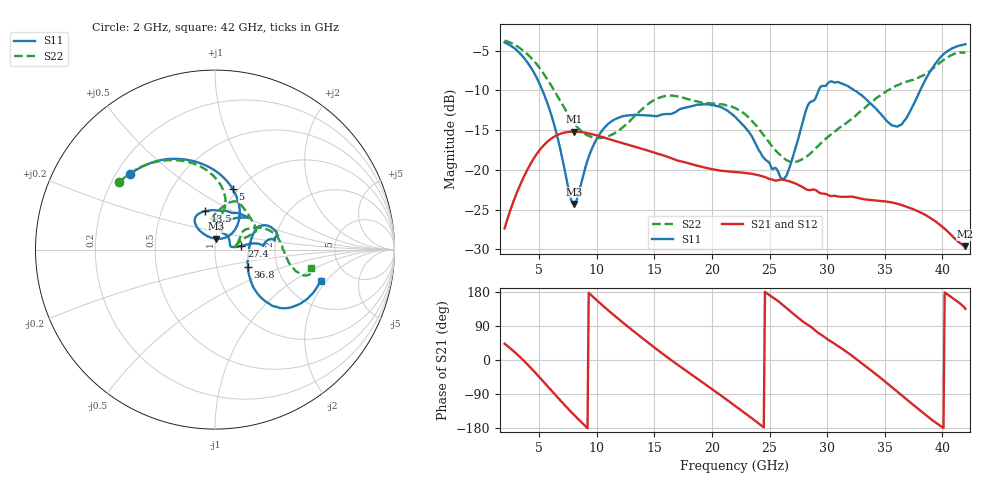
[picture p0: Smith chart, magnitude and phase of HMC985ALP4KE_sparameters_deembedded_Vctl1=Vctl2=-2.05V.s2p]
!s2p File: Measurements: S11, S21, S12, S22
# GHz S dB R 50.0
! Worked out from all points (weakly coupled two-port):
!   401 points, 2 GHz to 42 GHz, reference 50 ohm
!   highest |S21| = -15.18 dB at 8 GHz (marker M1); lowest = -29.6 dB at 42 GHz (marker M2)
!   lowest |S11| = -24.3 dB at 8 GHz (marker M3), VSWR 1.13, Z = 50.3 + j6.11 ohm
!   |S11| at or under -10 dB: 5.285 GHz to 29.26 GHz (23.98 GHz wide, 139 % of centre); 32.37 GHz to 38.07 GHz (5.705 GHz wide, 16.2 % of centre)
!   |S22| runs from -19.0 to -3.7 dB; largest |S21 - S12| = 0.00019
!   S11 on the Smith chart (normalised r, x): 2 GHz: 0.25, +0.36; 5 GHz: 0.94, +0.73; 13.5 GHz: 0.82, +0.37; 27.4 GHz: 1.34, +0.06; 36.8 GHz: 1.41, -0.29; 42 GHz: 3.16, -1.78
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2  -3.96 138.4  -27.37 42.9  -27.38 42.9  -3.72 144.9
3.5  -5.61 107.4  -21.40 3.0  -21.41 3.0  -4.87 119.6
5  -9.05 73.8  -17.59 -44.6  -17.59 -44.6  -7.10 95.5
6.6  -15.95 45.1  -15.61 -98.8  -15.61 -98.8  -10.75 78.5
8  -24.30 83.8  -15.18 -144.1  -15.19 -144.1  -14.04 79.9
8.7  -21.39 119.2  -15.26 -165.3  -15.26 -165.3  -15.18 86.2
10.6  -14.81 127.2  -15.92 141.4  -15.93 141.4  -15.93 100.1
13.5  -13.08 104.7  -17.17 68.7  -17.18 68.7  -12.95 83.3
15.4  -13.18 80.5  -18.02 23.9  -18.02 23.9  -10.93 70.2
18.9  -11.81 44.5  -19.54 -52.8  -19.55 -52.7  -11.45 44.9
22  -13.31 54.9  -20.27 -120.7  -20.28 -120.7  -12.22 23.5
24.5  -18.48 77.3  -20.86 -177.8  -20.86 -177.8  -15.64 20.1
26.1  -21.17 17.9  -21.24 146.5  -21.24 146.5  -18.38 11.7
27.4  -16.58 8.0  -21.82 113.4  -21.82 113.3  -18.97 8.3
28.7  -11.36 4.4  -22.49 84.9  -22.50 84.9  -17.70 15.7
29.5  -9.48 9.1  -22.97 66.2  -22.98 66.2  -16.58 23.2
31.1  -9.05 16.9  -23.38 33.7  -23.38 33.6  -14.67 33.0
33.3  -11.01 27.7  -23.72 -15.2  -23.73 -15.2  -12.16 29.3
35.4  -14.13 7.9  -24.06 -66.1  -24.05 -66.1  -9.90 19.6
36.8  -13.65 -28.1  -24.60 -101.5  -24.59 -101.4  -8.96 10.6
39.7  -6.06 -41.0  -26.80 -171.2  -26.81 -171.2  -6.63 -15.0
42  -4.18 -16.3  -29.60 134.9  -29.60 134.9  -5.24 -10.9
